FUNCTION_BLOCK p08_ST_spremljanjeMateriala
VAR_INPUT
END_VAR
VAR_OUTPUT
END_VAR
VAR
	lokacije: ARRAY[0..7] OF ST_LOCATION;
END_VAR

lokacije[0].occupied := TRUE;
lokacije[0].workpiece.id := 42;
lokacije[0].workpiece.recipe.directionMachine1 := FALSE;
lokacije[0].workpiece.recipe.timeMachine1 := T#1S;
lokacije[0].workpiece.recipe.positionSequence[0].rotation := 100;
lokacije[0].workpiece.recipe.positionSequence[0].lift := 50;
lokacije[0].workpiece.recipe.positionSequence[0].extension := 30;
lokacije[0].workpiece.recipe.positionSequence[0].grip := 15;

// Prenos materiala naprej
IF lokacije[0].isDone THEN
	lokacije[1].workpiece := lokacije[0].workpiece;
	lokacije[0].isDone := FALSE;
END_IF

END_FUNCTION_BLOCK
